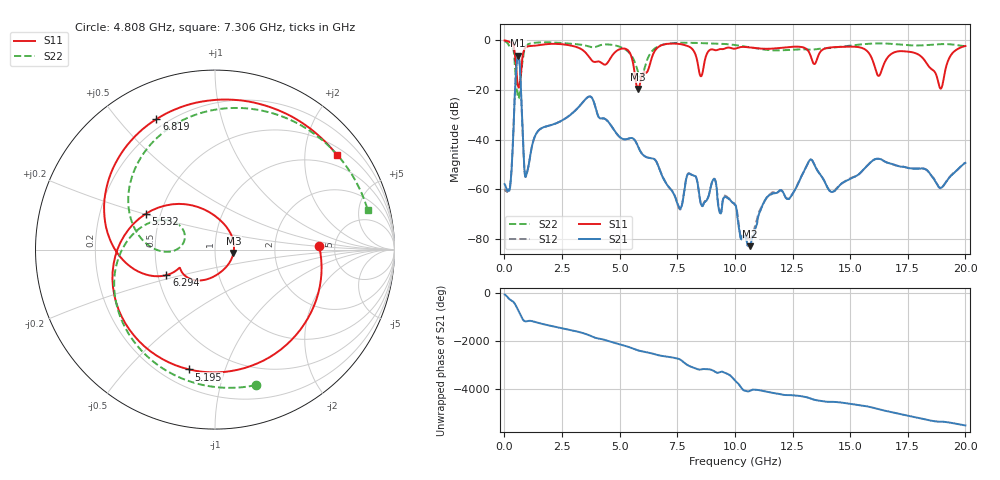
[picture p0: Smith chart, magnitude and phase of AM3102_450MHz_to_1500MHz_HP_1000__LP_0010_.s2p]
!Agilent Technologies,E8364B,MY43040894,A.07.50.67
!Agilent E8364B: A.07.50.67
!Date: Thursday, January 11, 2018 05:56:45
!Correction: S11(Full 2 Port(1,2))
!S21(Full 2 Port(1,2))
!S12(Full 2 Port(1,2))
!S22(Full 2 Port(1,2))
!S2P File: Measurements: S11, S21, S12, S22:
# Hz S  dB  R 50
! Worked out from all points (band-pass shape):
!   1601 points, 10 MHz to 20 GHz, reference 50 ohm
!   highest |S21| = -6.24 dB at 597.2 MHz (marker M1); lowest = -82.9 dB at 10.67 GHz (marker M2)
!   |S21| within 3 dB of the highest: 537.8 MHz to 661.2 MHz (123.3 MHz wide, 20.6 % of centre)
!   lowest |S11| = -19.6 dB at 5.795 GHz (marker M3), VSWR 1.23, Z = 61.4 - j2.41 ohm
!   |S11| at or under -10 dB: 5.599 GHz to 6.303 GHz (704.6 MHz wide, 11.8 % of centre); 16.05 GHz to 16.45 GHz (401.4 MHz wide, 2.47 % of centre); 18.37 GHz to 19.18 GHz (810.8 MHz wide, 4.32 % of centre)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
!   |S22| runs from -23.4 to -0.4 dB; largest |S21 - S12| = 0.0015
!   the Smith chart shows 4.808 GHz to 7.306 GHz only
!   S11 on the Smith chart (normalised r, x): 4.808 GHz: 3.75, +0.25; 5.195 GHz: 0.30, -0.76; 5.532 GHz: 0.41, +0.20; 6.294 GHz: 0.55, -0.17; 6.819 GHz: 0.16, +0.64; 7.306 GHz: 0.69, +2.78
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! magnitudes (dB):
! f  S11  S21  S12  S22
! 10 MHz  -0.1  -57.9  -60.3  -0.4
! 259.9 MHz  -0.8  -58.3  -57.6  -2.8
! 597.2 MHz  -18.6  -6.2  -6.2  -23.1
! 959.5 MHz  -2.6  -54.0  -54.0  -2.0
! 1.459 GHz  -2.0  -36.5  -36.6  -0.9
! 3.346 GHz  -3.6  -25.6  -25.6  -1.8
! 4.808 GHz  -4.7  -36.8  -36.8  -2.1
! 5.195 GHz  -3.3  -39.9  -39.9  -3.4
! 5.532 GHz  -7.2  -39.4  -39.4  -6.4
! 5.795 GHz  -19.6  -42.7  -42.7  -12.7
! 6.294 GHz  -10.3  -47.4  -47.4  -5.9
! 6.682 GHz  -2.7  -50.7  -50.8  -2.4
! 6.819 GHz  -2.0  -54.1  -54.0  -1.9
! 7.306 GHz  -1.3  -61.1  -61.0  -1.1
! 8.531 GHz  -14.5  -66.0  -66.1  -1.1
! 10.01 GHz  -3.4  -66.1  -66.2  -1.9
! 10.67 GHz  -2.9  -82.9  -79.8  -2.8
! 13.34 GHz  -7.8  -48.2  -48.2  -3.8
! 14.22 GHz  -2.8  -61.1  -61.0  -3.0
! 16.68 GHz  -6.3  -49.4  -49.4  -1.4
! 18.93 GHz  -19.5  -59.4  -59.6  -1.5
! 20 GHz  -2.3  -49.4  -49.3  -2.4
